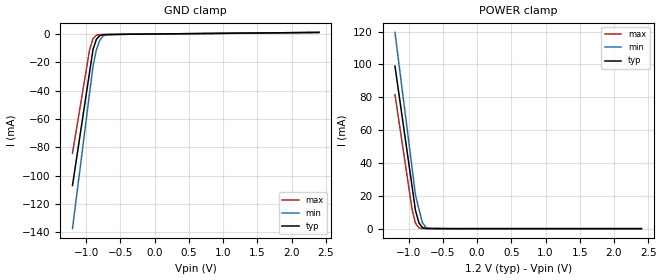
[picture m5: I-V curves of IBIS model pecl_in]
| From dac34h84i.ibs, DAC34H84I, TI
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[Model] pecl_in
Model_type Input
Vinl = 400.000mV
Vinh = 1.00000V
C_comp 876.000fF 875.000fF 877.000fF
| variable typ   min   max
[Voltage Range] 1.20000V 1.10000V 1.30000V
[POWER Clamp Reference] 1.20000V 1.10000V 1.30000V
[GND Clamp Reference] 0.00000V 0.00000V 0.00000V
[Temperature Range] 25   125   -40
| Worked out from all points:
|   GND clamp passes 1 mA (typ) near -0.79 V on its own axis
|   POWER clamp passes 1 mA (typ) near -0.81 V on its own axis
[GND Clamp]
-1.2V     -107.1mA   -137.5mA   -84.38mA
-950mV    -27mA      -41.87mA   -11.17mA
-900mV    -10.98mA   -22.74mA   -3.37mA
-850mV    -3.818mA   -11.06mA   -935.6uA
-800mV    -1.177mA   -4.383mA   -517.3uA
-750mV    -551.6uA   -1.488mA   -488.5uA
-700mV    -514.4uA   -633.4uA   -459.7uA
-650mV    -477.2uA   -431.8uA   -430.9uA
-400mV    -291.5uA   -281.3uA   -286.8uA
-375mV    -272.9uA   -266.2uA   -275.4uA
-325mV    -249.3uA   -236.1uA   -252.6uA
2.4V      1.033mA    1.033mA    989.7uA
[POWER Clamp]
-1.2V     98.97mA    119.5mA    81.62mA
-950mV    25.63mA    36.91mA    11.71mA
-900mV    10.96mA    20.38mA    3.296mA
-850mV    3.502mA    12.03mA    515.7uA
-800mV    708.3uA    3.676mA    54.89uA
-750mV    121.2uA    921.8uA    48.79uA
-650mV    88.9uA     30.96uA    36.59uA
2.4V      0A         0A         0A
